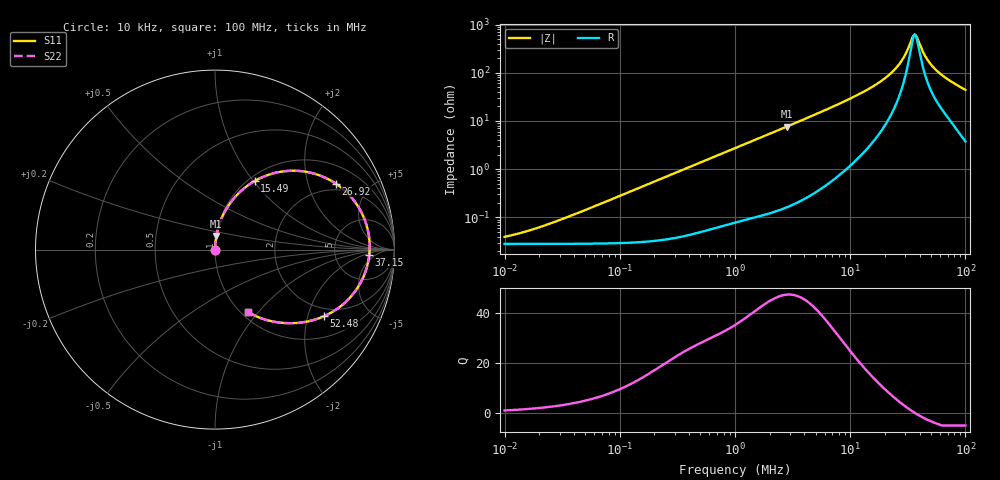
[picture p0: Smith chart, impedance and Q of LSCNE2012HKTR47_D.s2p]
! LSCNE2012HKTR47_D  S-PARAMETER MODEL  ( Standard Model )
! Model Generated by TAIYO YUDEN Corporation (http://www.ty-top.com)
! Version 1.0
! TAIYO YUDEN Control No. 210402
! Copyright(c) 2021 TAIYO YUDEN CO.,LTD. All Rights Reserved.
! Product Description (link to TY-COMPAS)
! https://ds.yuden.co.jp/TYCOMPAS/or/detail?pn=LSCNE2012HKTR47MD&u=M
! Products Name : Inductors
! Characteristics :
!  Inductance : 0.47 [uH] , SRF(min) : - [Hz] , DC Resistance(max) : 32 [mOhm]
!  Rated Current : Saturation  4.8 [A] (dL = 30 [%]), Temp Rise  4.0 [A] (dT = 40 [degC])
!  Case Size : 2.0 x 1.25 / 0.079 x 0.049 [mm/inch] , Thickness : 0.8 / 0.031 [mm/inch]
!  (Conditions: Temperature = 25 [degC] , DC Bias Current = 0 [A])
! External Node Assignments :
!  1  o---GGG---o  2
! GND o---------o GND
! Frequency Range : 10kHz  -  100MHz  [ 402 STEP ]
# MHz S RI R 50
! Freq[MHz].  S11 Real  S11 Imag  S21 Real  S21 Imag  S12 Real  S12 Imag  S22 Real  S22 Imag
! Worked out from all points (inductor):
!   401 points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, 10 kHz to 100 MHz, reference 50 ohm
!   read as one part in series: L = 441 nH near 30.9 kHz
!   highest Q = 47.2 at 2.818 MHz (marker M1), where L = 432 nH
!   self-resonance near 36.46 MHz
!   S11 on the Smith chart (normalised r, x): 10 kHz: 1.00, +0.00; 15.49 MHz: 1.07, +1.01; 26.92 MHz: 1.70, +3.04; 37.15 MHz: 13, -3; 52.48 MHz: 1.69, -2.54; 100 MHz: 1.08, -0.88
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0.01  0.000281 0.000277  0.9997 -0.000277  0.9997 -0.000277  0.000281 0.000277
0.019055  0.000282 0.000528  0.9997 -0.000528  0.9997 -0.000528  0.000282 0.000528
0.046774  0.000285 0.0013  0.9997 -0.0013  0.9997 -0.0013  0.000285 0.0013
0.218776  0.000369 0.00605  0.9996 -0.00605  0.9996 -0.00605  0.000369 0.00605
1  0.00152 0.0272  0.9985 -0.0272  0.9985 -0.0272  0.00152 0.0272
2.818383  0.0074 0.0758  0.9926 -0.0758  0.9926 -0.0758  0.0074 0.0758
4.677351  0.019 0.1253  0.981 -0.1253  0.981 -0.1253  0.019 0.1253
9.772372  0.083 0.2568  0.917 -0.2568  0.917 -0.2568  0.083 0.2568
12.58925  0.1414 0.3233  0.8586 -0.3233  0.8586 -0.3233  0.1414 0.3233
15.48817  0.2208 0.3818  0.7792 -0.3818  0.7792 -0.3818  0.2208 0.3818
18.62087  0.3288 0.4259  0.6712 -0.4259  0.6712 -0.4259  0.3288 0.4259
21.87762  0.4611 0.4387  0.5389 -0.4387  0.5389 -0.4387  0.4611 0.4387
26.91535  0.6736 0.3676  0.3264 -0.3676  0.3264 -0.3676  0.6736 0.3676
30.19952  0.7834 0.2611  0.2166 -0.2611  0.2166 -0.2611  0.7834 0.2611
34.67368  0.8579 0.0748  0.1421 -0.0748  0.1421 -0.0748  0.8579 0.0748
36.30781  0.8619 0.00585  0.1381 -0.00585  0.1381 -0.00585  0.8619 0.00585
37.15352  0.8597 -0.0285  0.1403 0.0285  0.1403 0.0285  0.8597 -0.0285
44.66836  0.7572 -0.2619  0.2428 0.2619  0.2428 0.2619  0.7572 -0.2619
52.48075  0.6071 -0.3714  0.3929 0.3714  0.3929 0.3714  0.6071 -0.3714
60.25596  0.4841 -0.4057  0.5159 0.4057  0.5159 0.4057  0.4841 -0.4057
72.4436  0.3493 -0.4053  0.6507 0.4053  0.6507 0.4053  0.3493 -0.4053
100  0.1833 -0.3466  0.8167 0.3466  0.8167 0.3466  0.1833 -0.3466
